|Texas Instruments Incorporated
| MULTI-CHANNEL HIGH SPEED ADC WITH JESD204B INTERFACE
| part#   Digital Voltage Range   Package-type   #pins
| ADS52J90   1.7V - 1.9V   BGA   198
[IBIS Ver]   4.1
[File name]   ads52j90.ibs
[File Rev]   1.0
[Date]   12/08/2014
[Source]
| Texas Instruments Incorporated.
| Analog-eLab Design Center, HPA
| 12500 TI Blvd
| Dallas, TX -75243
[Notes]   Revision History:
| Rev 1.0: 12/08/2014
| - Initial version of the model
| - Model generated from simulations in TISPICE
| - C_comp although listed in numerical order of value are
|   obtained from varying PVT conditions. For PVT conditions for
|   each specific value refer the buffer description under
|   respective [Model]. IBIS model user is responsible for using
|   appropriate C_comp to simulate for Signal Integrity.
[Disclaimer]
| This model is designed as an aid for customers of Texas Instruments.
| TI and its licensors and suppliers make no warranties, either expressed
| or implied, with respect to this  model, including the warranties of
| merchantability or fitness for a particular purpose. The model is
| provided solely on an "as is" basis. The entire risk as to its quality
| and performance is with the customer.
[Copyright]
 (C) Copyright 2014 Texas Instruments Incorporated.All rights reserved.
|   Device
[Component]   ADS52J90
[Manufacturer]   TI
[Package]
|   typ   min   max
R_pkg  1.000E-02   0.800E-02   1.200E-02
L_pkg  1.602E-09   1.280E-09   1.920E-09
C_pkg  0.700E-13   0.560E-13   0.840E-12
[Pin]  signal_name   model_name   R_pin   L_pin   C_pin
A1   INM2   NC   NA   NA   NA
A2   INP2   NC   NA   NA   NA
A3   INP1   NC   NA   NA   NA
A4   AVDD   POWER   NA   NA   NA
A5   SDATA   SCLK_INPUT   NA   NA   NA
A6   RESET   SCLK_INPUT   NA   NA   NA
A7   DVDD   POWER   NA   NA   NA
A8   DVSS   GND   NA   NA   NA
A9   CML1_OUTP   CML_OUT   NA   NA   NA
A10   CML1OUTM   CML_OUT   NA   NA   NA
A11   CML2_OUTP   CML_OUT   NA   NA   NA
B1   INM3   NC   NA   NA   NA
B2   INP3   NC   NA   NA   NA
B3   INM1   NC   NA   NA   NA
B4   AVSS   GND   NA   NA   NA
B5   SEN   SEN   NA   NA   NA
B6   RESEVED_DIGITAL_PIN   NC   NA   NA   NA
B7   SCLK   SCLK_INPUT   NA   NA   NA
B8   DVDD   POWER   NA   NA   NA
B9   DOUTP1   LVDS_OUT   NA   NA   NA
B10   DOUTM1   LVDS_OUT   NA   NA   NA
B11   CML2_OUTM   CML_OUT   NA   NA   NA
C1   INM5   NC   NA   NA   NA
C2   INP5   NC   NA   NA   NA
C3   INP4   NC   NA   NA   NA
C4   AVSS   GND   NA   NA   NA
C5   SDOUT   SDOUT   NA   NA   NA
C6   PND_FAST   SCLK_INPUT   NA   NA   NA
C7   PDN_GBL   SCLK_INPUT   NA   NA   NA
C8   DVDD   POWER   NA   NA   NA
C9   DOUTP2   LVDS_OUT   NA   NA   NA
C10   DOUTM2   LVDS_OUT   NA   NA   NA
C11   CML3_OUTP   CML_OUT   NA   NA   NA
D1   INM6   NC   NA   NA   NA
D2   INP6   NC   NA   NA   NA
D3   INM4   NC   NA   NA   NA
D4   AVSS   GND   NA   NA   NA
D5   NC   NC   NA   NA   NA
D6   SNYC   SEN   NA   NA   NA
D7   DVSS   GND   NA   NA   NA
D8   DVDD   POWER   NA   NA   NA
D9   DOUTP3   LVDS_OUT   NA   NA   NA
D10   DOUTM3   LVDS_OUT   NA   NA   NA
D11   CML3_OUTM   CML_OUT   NA   NA   NA
E1   INM7   NC   NA   NA   NA
E2   INP7   NC   NA   NA   NA
E3   INM8   NC   NA   NA   NA
E4   INP8   NC   NA   NA   NA
E5   VREF_IN   NC   NA   NA   NA
E6   AVDD   POWER   NA   NA   NA
E7   DVSS   GND   NA   NA   NA
E8   LVDD   POWER   NA   NA   NA
E9   DOUTP4   LVDS_OUT   NA   NA   NA
E10   DOUTM4   LVDS_OUT   NA   NA   NA
E11   CML4_OUTP   CML_OUT   NA   NA   NA
F1   INM9   NC   NA   NA   NA
F2   INP9   NC   NA   NA   NA
F3   INM10   NC   NA   NA   NA
F4   INP10   NC   NA   NA   NA
F5   VCM   NC   NA   NA   NA
F6   AVDD   POWER   NA   NA   NA
F7   DVDD   POWER   NA   NA   NA
F8   LVDD   POWER   NA   NA   NA
F9   DOUTP5   LVDS_OUT   NA   NA   NA
F10   DOUTM5   LVDS_OUT   NA   NA   NA
F11   CML4_OUTM   CML_OUT   NA   NA   NA
G1   INM11   NC   NA   NA   NA
G2   INP11   NC   NA   NA   NA
G3   INM12   NC   NA   NA   NA
G4   INP12   NC   NA   NA   NA
G5   AVDD   POWER   NA   NA   NA
G6   AVDD   POWER   NA   NA   NA
G7   DVDD   POWER   NA   NA   NA
G8   LVDD   POWER   NA   NA   NA
G9   DOUTP6   LVDS_OUT   NA   NA   NA
G10   DOUTM6   LVDS_OUT   NA   NA   NA
G11   DOUTM8   LVDS_OUT   NA   NA   NA
H1   INM13   NC   NA   NA   NA
H2   INP13   NC   NA   NA   NA
H3   INM14   NC   NA   NA   NA
H4   INP14   NC   NA   NA   NA
H5   AVSS   GND   NA   NA   NA
H6   AVSS   GND   NA   NA   NA
H7   DVSS   GND   NA   NA   NA
H8   DVSS   GND   NA   NA   NA
H9   DOUTP7   LVDS_OUT   NA   NA   NA
H10   DOUTM7   LVDS_OUT   NA   NA   NA
H11   DOUTP8   LVDS_OUT   NA   NA   NA
J1   INM15   NC   NA   NA   NA
J2   INP15   NC   NA   NA   NA
J3   INM16   NC   NA   NA   NA
J4   INP16   NC   NA   NA   NA
J5   AVSS   GND   NA   NA   NA
J6   AVSS   GND   NA   NA   NA
J7   DVSS   GND   NA   NA   NA
J8   DVSS   GND   NA   NA   NA
J9   FCLKP   LVDS_OUT   NA   NA   NA
J10   LVDD   POWER   NA   NA   NA
J11   DCLKP   LVDS_OUT   NA   NA   NA
K1   INM17   NC   NA   NA   NA
K2   INP17   NC   NA   NA   NA
K3   INM18   NC   NA   NA   NA
K4   INP18   NC   NA   NA   NA
K5   AVSS   GND   NA   NA   NA
K6   AVSS   GND   NA   NA   NA
K7   DVSS   GND   NA   NA   NA
K8   DVSS   GND   NA   NA   NA
K9   FCLKM   LVDS_OUT   NA   NA   NA
K10   DVSS   GND   NA   NA   NA
K11   DCLKM   LVDS_OUT   NA   NA   NA
L1   INM19   NC   NA   NA   NA
L2   INP19   NC   NA   NA   NA
L3   INM20   NC   NA   NA   NA
L4   INP20   NC   NA   NA   NA
L5   AVSS   GND   NA   NA   NA
L6   AVSS   GND   NA   NA   NA
L7   DVSS   GND   NA   NA   NA
L8   DVSS   GND   NA   NA   NA
L9   DOUTP10   LVDS_OUT   NA   NA   NA
L10   DOUTM10   LVDS_OUT   NA   NA   NA
L11   DOUTP9   LVDS_OUT   NA   NA   NA
M1   INM21   NC   NA   NA   NA
M2   INP21   NC   NA   NA   NA
M3   INM22   NC   NA   NA   NA
M4   INP22   NC   NA   NA   NA
M5   AVDD   POWER   NA   NA   NA
M6   AVDD   POWER   NA   NA   NA
M7   DVDD   POWER   NA   NA   NA
M8   LVDD   POWER   NA   NA   NA
M9   DOUTP11   LVDS_OUT   NA   NA   NA
M10   DOUTM11   LVDS_OUT   NA   NA   NA
M11   DOUTM9   LVDS_OUT   NA   NA   NA
N1   INM23   NC   NA   NA   NA
N2   INP23   NC   NA   NA   NA
N3   INM24   NC   NA   NA   NA
N4   INP24   NC   NA   NA   NA
N5   NC   NC   NA   NA   NA
N6   AVDD   POWER   NA   NA   NA
N7   DVDD   POWER   NA   NA   NA
N8   LVDD   POWER   NA   NA   NA
N9   DOUTP12   LVDS_OUT   NA   NA   NA
N10   DOUTM12   LVDS_OUT   NA   NA   NA
N11   CML8_OUTM   CML_OUT   NA   NA   NA
P1   INM25   NC   NA   NA   NA
P2   INP25   NC   NA   NA   NA
P3   INM26   NC   NA   NA   NA
P4   INP26   NC   NA   NA   NA
P5   NC   NC   NA   NA   NA
P6   AVDD   POWER   NA   NA   NA
P7   SYNCM_SERDES   SYNC_INPUT   NA   NA   NA
P8   LVDD   POWER   NA   NA   NA
P9   DOUTP13   LVDS_OUT   NA   NA   NA
P10   DOUTM13   LVDS_OUT   NA   NA   NA
P11   CML8_OUTP   CML_OUT   NA   NA   NA
R1   NIM27   NC   NA   NA   NA
R2   INP27   NC   NA   NA   NA
R3   INM28   NC   NA   NA   NA
R4   AVSS   GND   NA   NA   NA
R5   AVSS   GND   NA   NA   NA
R6   DVSS   GND   NA   NA   NA
R7   SYNCP_SERDES   SYNC_INPUT   NA   NA   NA
R8   DVDD   POWER   NA   NA   NA
R9   DOUTP14   LVDS_OUT   NA   NA   NA
R10   DOUTM14   LVDS_OUT   NA   NA   NA
R11   CML7_OUTM   CML_OUT   NA   NA   NA
T1   INM29   NC   NA   NA   NA
T2   INP29   NC   NA   NA   NA
T3   INP28   NC   NA   NA   NA
T4   AVSS   GND   NA   NA   NA
T5   AVSS   GND   NA   NA   NA
T6   DVDD   POWER   NA   NA   NA
T7   SYSREFM_SERDES   SYNC_INPUT   NA   NA   NA
T8   DVDD   POWER   NA   NA   NA
T9   DOUTP15   LVDS_OUT   NA   NA   NA
T10   DOUTM15   LVDS_OUT   NA   NA   NA
T11   CML7_OUTP   CML_OUT   NA   NA   NA
U1   INM30   NC   NA   NA   NA
U2   INP30   NC   NA   NA   NA
U3   INM32   NC   NA   NA   NA
U4   AVSS   GND   NA   NA   NA
U5   CLKM   CLK_INPUT   NA   NA   NA
U6   AVSS   GND   NA   NA   NA
U7   SYSREFP_SERDES   SYNC_INPUT   NA   NA   NA
U8   DVDD   POWER   NA   NA   NA
U9   DOUTP16   LVDS_OUT   NA   NA   NA
U10   DOUTM16   LVDS_OUT   NA   NA   NA
U11   CML6_OUTM   CML_OUT   NA   NA   NA
V1   INM31   NC   NA   NA   NA
V2   INP31   NC   NA   NA   NA
V3   INP32   NC   NA   NA   NA
V4   AVDD   POWER   NA   NA   NA
V5   CLKP   CLK_INPUT   NA   NA   NA
V6   AVSS   GND   NA   NA   NA
V7   DVDD   POWER   NA   NA   NA
V8   DVSS   GND   NA   NA   NA
V9   CML5_OUTP   CML_OUT   NA   NA   NA
V10   CML5_OUTM   CML_OUT   NA   NA   NA
V11   CML6_OUTP   CML_OUT   NA   NA   NA
[Diff Pin]  inv_pin  vdiff  tdelay_typ tdelay_min tdelay_max
A9   A10   NA   NA   NA   NA
A11   B11   NA   NA   NA   NA
C11   D11   NA   NA   NA   NA
E11   F11   NA   NA   NA   NA
P11   N11   NA   NA   NA   NA
T11   R11   NA   NA   NA   NA
V11   U11   NA   NA   NA   NA
V9   V10   NA   NA   NA   NA
B9   B10   NA   NA   NA   NA
C9   C10   NA   NA   NA   NA
D9   D10   NA   NA   NA   NA
E9   E10   NA   NA   NA   NA
F9   F10   NA   NA   NA   NA
G9   G10   NA   NA   NA   NA
H9   H10   NA   NA   NA   NA
L9   L10   NA   NA   NA   NA
M9   M10   NA   NA   NA   NA
N9   N10   NA   NA   NA   NA
P9   P10   NA   NA   NA   NA
R9   R10   NA   NA   NA   NA
T9   T10   NA   NA   NA   NA
U9   U10   NA   NA   NA   NA
H11   G11   NA   NA   NA   NA
L11   M11   NA   NA   NA   NA
V5   U5   NA   NA   NA   NA
R7   P7   NA   NA   NA   NA
U7   T7   NA   NA   NA   NA
J9   K9   NA   NA   NA   NA
J11   K11   NA   NA   NA   NA
| Models and submodels in the file (7): CML_OUT (Output), LVDS_OUT (Output), SDOUT (Output), SYNC_INPUT (Input), SEN (Input), SCLK_INPUT (Input), CLK_INPUT (Input)
